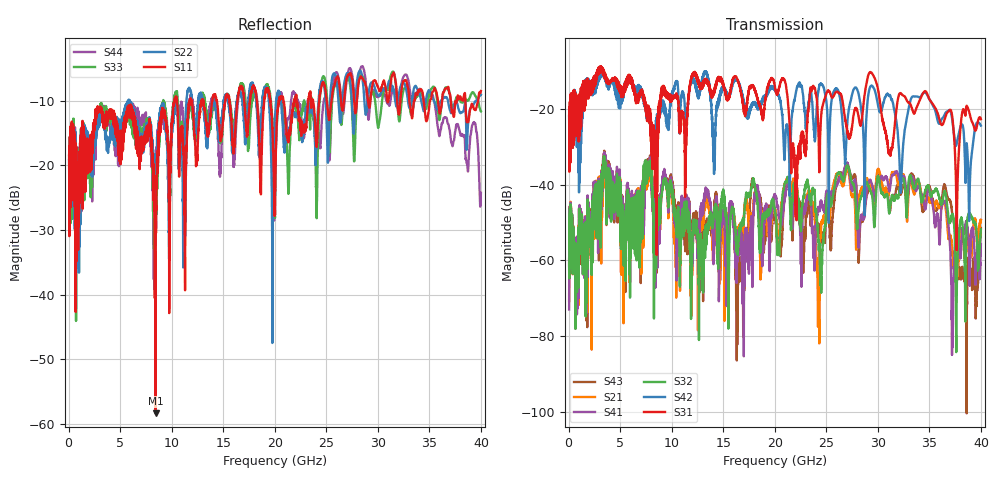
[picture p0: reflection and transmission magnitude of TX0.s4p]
!Agilent Technologies,N5245A,MY49151084,A.09.00.04
!Agilent N5245A: A.09.00.04
!Date: Thursday, January 20, 2011 08:43:31
!Correction: S11(Full 4 Port(1,2,3,4))
!S12(Full 4 Port(1,2,3,4))
!S13(Full 4 Port(1,2,3,4))
!S14(Full 4 Port(1,2,3,4))
!S21(Full 4 Port(1,2,3,4))
!S22(Full 4 Port(1,2,3,4))
!S23(Full 4 Port(1,2,3,4))
!S24(Full 4 Port(1,2,3,4))
!S31(Full 4 Port(1,2,3,4))
!S32(Full 4 Port(1,2,3,4))
!S33(Full 4 Port(1,2,3,4))
!S34(Full 4 Port(1,2,3,4))
!S41(Full 4 Port(1,2,3,4))
!S42(Full 4 Port(1,2,3,4))
!S43(Full 4 Port(1,2,3,4))
!S44(Full 4 Port(1,2,3,4))
!S4P File: Measurements: <S11,S12,S13,S14>,
!<S21,S22,S23,S24>,
!<S31,S32,S33,S34>,
!<S41,S42,S43,S44>:
# Hz S  dB  R 50
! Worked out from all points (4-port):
!   3996 points, 50 MHz to 40 GHz, reference 50 ohm
!   strongest paths, dB at 50 MHz, 10.04 GHz, 20.03 GHz, 30.02 GHz, 40 GHz:
!     S31: -21.9, -17.0, -14.4, -14.9, -22.7
!     S42: -22.3, -15.6, -15.0, -19.1, -24.4
!     S32: -60.8, -41.5, -47.2, -37.8, -51.8
!     S41: -73.0, -40.7, -42.7, -38.6, -55.7
!     S21: -70.7, -42.3, -46.4, -35.9, -49.2
!     S43: -59.6, -39.7, -48.5, -36.8, -51.4
!   lowest |S11| = -58.3 dB at 8.44 GHz (marker M1), VSWR 1.00, Z = 50.1 + j0.0787 ohm
!   |S11| at or under -10 dB: start of sweep to 10.26 GHz; 10.52 GHz to 11.77 GHz (1.255 GHz wide, 11.3 % of centre); 38.49 GHz to 39.74 GHz (1.245 GHz wide, 3.18 % of centre)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
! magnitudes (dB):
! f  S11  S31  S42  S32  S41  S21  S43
! 50 MHz  -18.4  -21.9  -22.3  -60.8  -73.0  -70.7  -59.6
! 3.45 GHz  -14.0  -11.3  -11.1  -33.3  -33.0  -34.8  -31.5
! 8.44 GHz  -58.3  -27.9  -24.7  -59.7  -48.4  -48.8  -50.0
! 21.89 GHz  -10.0  -32.4  -17.8  -39.9  -42.2  -39.1  -43.6
! 24.19 GHz  -13.2  -22.8  -15.9  -52.2  -46.4  -73.7  -50.8
! 26.98 GHz  -6.5  -24.8  -26.4  -35.3  -34.2  -36.0  -34.6
! 40 GHz  -8.5  -22.7  -24.4  -51.8  -55.7  -49.2  -51.4
